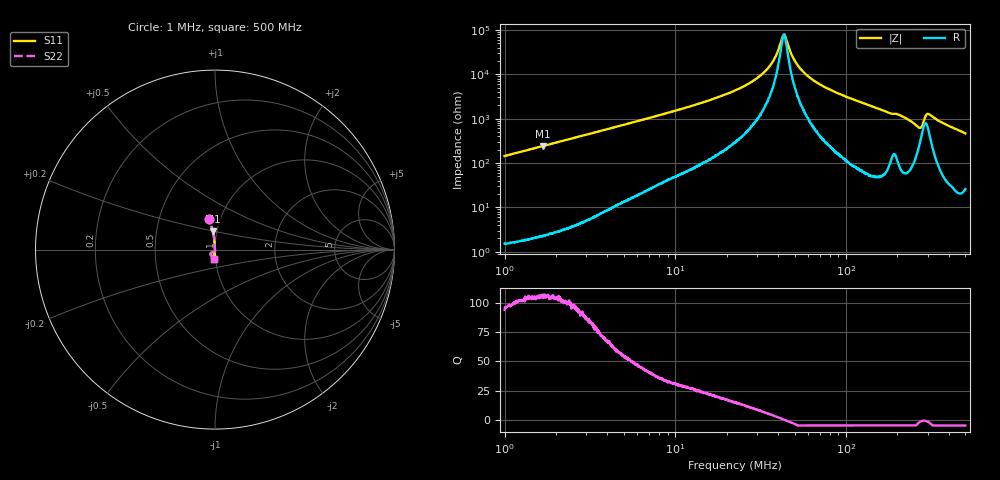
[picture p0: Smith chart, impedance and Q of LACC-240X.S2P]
!s-Parameter Generated by FASTRON Sdn. Bhd.
!FASTRON P/N : LACC-240X
!Keysight Technologies,E4991B,MY54100416,A.01.15
!Date: Wed Mar 18 09:37:50 2026
!Version  : Rev00 Wed Mar 18 09:37:50 2026
!Data & Calibration Information:
!PortZ  Port1:50+j0  Port2:50+j0
!When reading, reference impedance value at option line is always used.
!Remarks : This data is being provided solely for informational purposes.
!Freq	S11	S21	S12	S22
# Hz S dB R 50
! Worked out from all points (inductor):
!   1601 points, 1 MHz to 500 MHz, reference 50 ohm
!   read as one part in shunt: L = 22.8 uH near 1.032 MHz
!   highest Q = 106 at 1.676 MHz (marker M1), where L = 22.9 uH
!   self-resonance near 43.28 MHz
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1000000  -15.33 100.5  -0.15 9.9  -0.15 9.9  -15.33 100.5
1676301  -19.73 96.5  -0.05 5.9  -0.05 5.9  -19.73 96.5
2820919  -24.25 94.1  -0.02 3.5  -0.02 3.5  -24.25 94.1
7957584  -33.46 92.8  -0.01 1.2  -0.01 1.2  -33.46 92.8
2.236068e7  -44.70 94.2  -0.00 0.3  -0.00 0.3  -44.70 94.2
2.878264e7  -49.22 96.1  -0.00 0.2  -0.00 0.2  -49.22 96.1
3.427987e7  -54.09 100.3  -0.00 0.1  -0.00 0.1  -54.09 100.3
3.821828e7  -59.35 108.5  -0.00 0.1  -0.00 0.1  -59.35 108.5
4.227946e7  -68.41 151.3  -0.00 0.0  -0.00 0.0  -68.41 151.3
4.327634e7  -69.81 178.2  -0.00 0.0  -0.00 0.0  -69.81 178.2
4.429673e7  -68.68 -148.7  -0.00 -0.0  -0.00 -0.0  -68.68 -148.7
4.7875e7  -60.91 -110.5  -0.00 -0.0  -0.00 -0.0  -60.91 -110.5
5.134194e7  -56.81 -102.7  -0.00 -0.1  -0.00 -0.1  -56.81 -102.7
6.307767e7  -49.78 -95.5  -0.00 -0.2  -0.00 -0.2  -49.78 -95.5
8.912629e7  -43.54 -92.9  -0.00 -0.4  -0.00 -0.4  -43.54 -92.9
1.77937e8  -34.68 -94.6  -0.01 -1.1  -0.01 -1.1  -34.68 -94.6
2.078454e8  -33.49 -94.8  -0.01 -1.2  -0.01 -1.2  -33.49 -94.8
2.685796e8  -28.04 -116.0  -0.15 -2.1  -0.15 -2.1  -28.04 -116.0
2.770562e8  -28.58 -131.6  -0.21 -1.6  -0.21 -1.6  -28.58 -131.6
2.948204e8  -33.82 -130.4  -0.11 -0.9  -0.11 -0.9  -33.82 -130.4
3.053088e8  -34.15 -114.4  -0.07 -1.0  -0.07 -1.0  -34.15 -114.4
5e8  -25.41 -96.3  -0.04 -3.1  -0.04 -3.1  -25.41 -96.3
